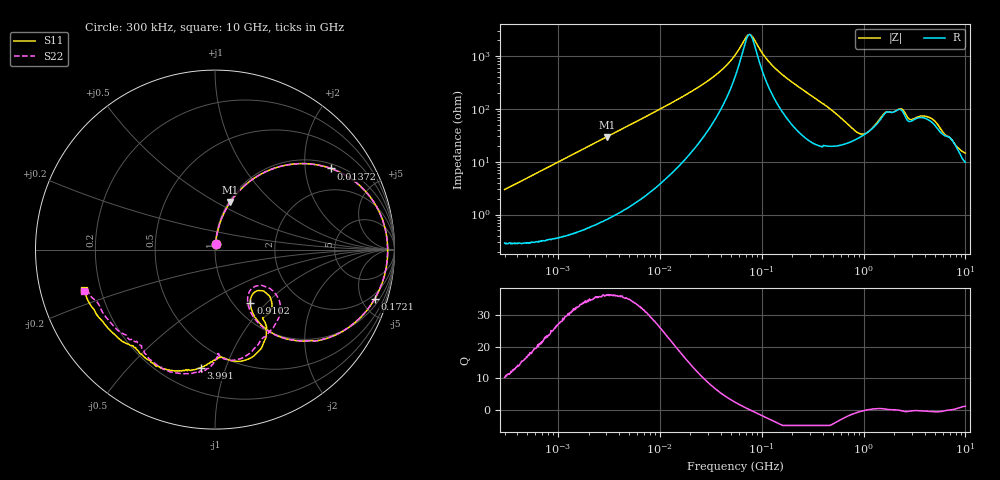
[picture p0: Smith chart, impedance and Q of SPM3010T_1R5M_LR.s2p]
! S-Parameter Data Generated by TDK Corporation
! Copyright(C) 2019 TDK Corporation.
! All Rights Reserved.
! TDK P/N: SPM3010T-1R5M-LR (Inductor)
! Property: L=1.5uH at 100kHz
! Size(LxWxT): 3.2x3x1mm
! Model Type: s2p (Touchstone File Format Version 1.0)
! Frequency: DC=Yes Start=0.3MHz Stop=10000MHz 802points Log-sweep
! Model Generated on Sep. 23, 2019
! Port Assignments:
!  1 ---@@@--- 2
! Applicable Conditions:
!  Temperature = 25 degC
!  DC Bias Current = 0 A
!  Small Signal Operation
! Terms and conditions regarding TDK Simulation Models
! (1)This simulation model is being provided solely for informational purposes. Please refer to the specifications of the products in terms of detailed characteristics of such products.
! (2)In no event shall TDK Corporation of any of its subsidiaries be liable for any loss or damage arising, directly or indirectly,
!  From any information contained in this simulation model, including, but not limited to loss or damages arising from any inaccuracies, omissions or errors in connection with such information.
! (3)Any and all copyrights on this simulation model are owned by TDK Corporation.
!  Duplication or redistribution of this simulation model without prior written permission from TDK Corporation is prohibited.
! (4)This simulation model is subject to any modification or change without any prior notice.
! (5)Neither TDK Corporation nor any of its subsidiaries shall make any warranty, express or implied,
!  Including but not limited to the correctness, implied warranties of merchantability and fitness for a particular purpose with respect to this simulation models.
! (6)The use of this simulation model shall be deemed to have consented to the terms and conditions hereof.
# Hz S MA R 50
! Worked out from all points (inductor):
!   801 points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, 300 kHz to 10 GHz, reference 50 ohm
!   read as one part in series: L = 1.56 uH near 318.3 kHz
!   highest Q = 36.4 at 3.017 MHz (marker M1), where L = 1.55 uH
!   self-resonance near 76.11 MHz
!   S11 on the Smith chart (normalised r, x): 300 kHz: 1.01, +0.06; 13.72 MHz: 1.15, +2.73; 172.1 MHz: 1.50, -6.22; 910.2 MHz: 1.19, -0.81; 3.991 GHz: 0.35, -0.82; 10 GHz: 0.14, -0.15
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300000  0.03036 82.8  0.9967 -1.7  0.9966 -1.6  0.03032 83.0
1713600  0.164 78.8  0.9815 -9.4  0.9815 -9.4  0.1639 78.9
3016998  0.2788 72.2  0.9526 -16.2  0.9529 -16.2  0.2788 72.2
5292453  0.4507 61.5  0.8796 -26.9  0.8799 -26.9  0.4507 61.5
9671944  0.6737 45.3  0.714 -42.5  0.7145 -42.5  0.6736 45.3
1.372114e7  0.7876 35.1  0.5792 -52.2  0.5796 -52.2  0.7875 35.0
3.162388e7  0.9354 13.9  0.2548 -68.8  0.2549 -68.8  0.9351 13.9
5.477226e7  0.9601 3.7  0.0937 -63.5  0.09377 -63.5  0.9596 3.7
7.683413e7  0.9622 -1.9  0.03812 1.8  0.03814 1.8  0.9616 -1.9
1.161426e8  0.9546 -9.1  0.1189 61.5  0.119 61.5  0.9538 -9.1
1.720721e8  0.9309 -17.3  0.235 62.4  0.2351 62.4  0.9297 -17.3
3.126428e8  0.8308 -34.4  0.4608 48.3  0.461 48.3  0.8288 -34.5
5.165633e8  0.6334 -51.5  0.6528 26.7  0.653 26.7  0.6291 -51.8
9.101824e8  0.358 -56.6  0.7367 -4.6  0.737 -4.6  0.3435 -58.0
1.133369e9  0.3245 -46.6  0.7002 -17.5  0.7004 -17.5  0.2985 -47.0
1.371335e9  0.3722 -40.4  0.6233 -28.8  0.6235 -28.8  0.3385 -36.8
1.767019e9  0.4644 -53.2  0.4812 -31.2  0.4813 -31.2  0.5238 -47.9
2.264206e9  0.5703 -60.4  0.4184 -33.1  0.4187 -33.1  0.6051 -70.4
2.598782e9  0.6388 -75.6  0.4485 -27.6  0.4486 -27.6  0.6138 -84.5
3.991169e9  0.6628 -96.9  0.3973 -45.4  0.3974 -45.4  0.6843 -95.9
5.687864e9  0.7224 -118.2  0.4058 -52.4  0.4058 -52.5  0.7159 -118.5
1e10  0.7609 -162.9  0.3365 -95.0  0.3371 -95.3  0.7672 -162.5
